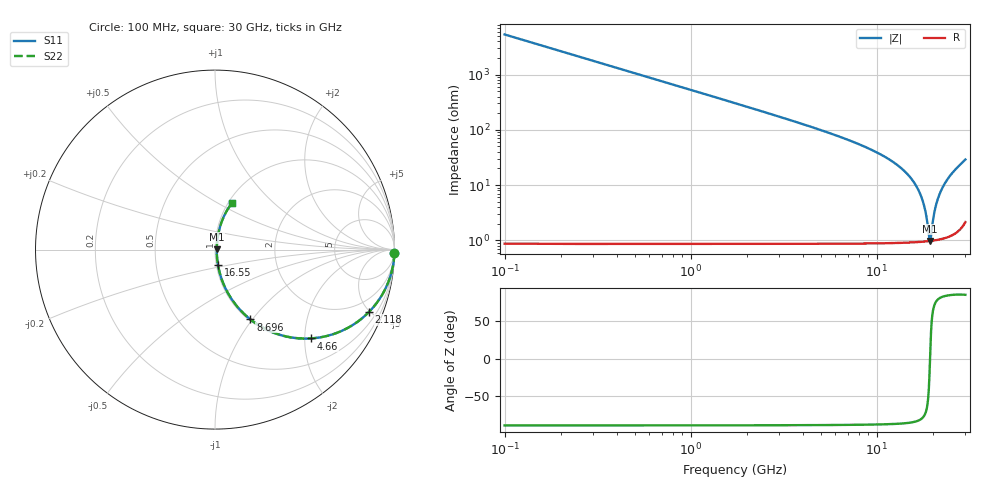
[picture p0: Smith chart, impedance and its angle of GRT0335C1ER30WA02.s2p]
!Murata Part Number: GRT0335C1ER30WA02
!These Parameters are Measured in Series Mode Connection
!Data Generated on Jun 19, 2026
!  o--ll--o
!Port1  Port2
!  o------o
!Operation Temp=25[degC], DC Bias Voltage=0[V]
!Freq. Start=100[MHz] Stop=30[GHz] 401[Steps]
# Hz S RI R 50
!Freq.(Hz) S11(Real) S11(Imag) S21(Real) S21(Imag) S12(Real) S12(Imag) S22(Real) S22(Imag)
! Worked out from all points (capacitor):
!   401 points, 100 MHz to 30 GHz, reference 50 ohm
!   read as one part in series: C = 300 fF near 249.5 MHz
!   lowest |Z| = 979 mohm at 19.39 GHz (marker M1)
!   series resonance near 19.36 GHz, so ESL is about 230 pH
!   S11 on the Smith chart (normalised r, x): 100 MHz: open; 2.118 GHz: 1.02, -4.95; 4.66 GHz: 1.02, -2.15; 8.696 GHz: 1.02, -0.98; 16.55 GHz: 1.02, -0.18; 30 GHz: 1.04, +0.58
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1e8  0.9996 -0.0188  0.000358 0.0188  0.000358 0.0188  0.9996 -0.0188
3.99e8  0.9943 -0.0748  0.00568 0.0748  0.00568 0.0748  0.9943 -0.0748
7.7275e8  0.979 -0.1428  0.021 0.1428  0.021 0.1428  0.979 -0.1428
1.37075e9  0.9364 -0.243  0.0636 0.243  0.0636 0.243  0.9364 -0.243
2.11825e9  0.8588 -0.3465  0.1412 0.3465  0.1412 0.3465  0.8588 -0.3465
3.2395e9  0.7163 -0.4481  0.2837 0.4481  0.2837 0.4481  0.7163 -0.4481
4.65975e9  0.5354 -0.4947  0.4646 0.4947  0.4646 0.4947  0.5354 -0.4947
5.10825e9  0.4839 -0.4953  0.5161 0.4953  0.5161 0.4953  0.4839 -0.4953
8.69625e9  0.1977 -0.3894  0.8023 0.3894  0.8023 0.3894  0.1977 -0.3894
1.01165e10  0.1342 -0.3296  0.8658 0.3296  0.8658 0.3296  0.1342 -0.3296
1.505e10  0.0283 -0.1368  0.9717 0.1368  0.9717 0.1368  0.0283 -0.1368
1.6545e10  0.0168 -0.0862  0.9832 0.0862  0.9832 0.0862  0.0168 -0.0862
1.811475e10  0.0108 -0.0369  0.9892 0.0369  0.9892 0.0369  0.0108 -0.0369
1.8638e10  0.00999 -0.0212  0.99 0.0212  0.99 0.0212  0.00999 -0.0212
1.916125e10  0.00967 -0.00586  0.9903 0.00586  0.9903 0.00586  0.00967 -0.00586
1.93855e10  0.00968 0.000603  0.9903 -0.000603  0.9903 -0.000603  0.00968 0.000603
2.005825e10  0.0102 0.0196  0.9898 -0.0196  0.9898 -0.0196  0.0102 0.0196
2.080575e10  0.0116 0.0401  0.9884 -0.0401  0.9884 -0.0401  0.0116 0.0401
2.17775e10  0.0147 0.0659  0.9853 -0.0659  0.9853 -0.0659  0.0147 0.0659
2.319775e10  0.0214 0.1019  0.9786 -0.1019  0.9786 -0.1019  0.0214 0.1019
2.50665e10  0.0342 0.1468  0.9658 -0.1468  0.9658 -0.1468  0.0342 0.1468
3e10  0.0938 0.2569  0.9062 -0.2569  0.9062 -0.2569  0.0938 0.2569
